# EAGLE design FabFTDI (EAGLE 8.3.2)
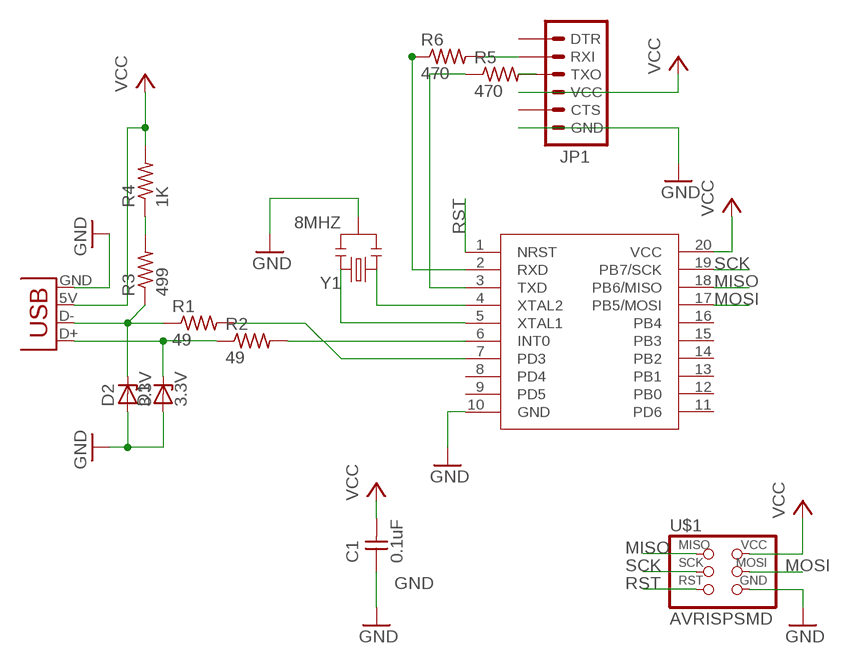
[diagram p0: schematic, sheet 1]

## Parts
C1  0.1uF  UNPOLARIZED_CAPACITOR1206  [1206]
D1  3.3V  ZENER_DIODESOD123  [SOD123]
D2  3.3V  ZENER_DIODESOD123  [SOD123]
JP1  FTDI_CONNECTORSMD  [1X06-SMD]
JP2  USBPCB  [USB_PCB]
R1  49  RESISTOR1206  [1206]
R2  49  RESISTOR1206  [1206]
R3  499  RESISTOR1206  [1206]
R4  1K  RESISTOR1206  [1206]
R5  470  RESISTOR1206  [1206]
R6  470  RESISTOR1206  [1206]
U$1  AVRISPSMD  [2X03SMD]
U$2  ATTINY2313  [SO20W]
Y1  8MHZ  RESONATOR8MHZ  [RESONATOR-SMD]

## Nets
GND: C1.1 D1.ANODE D2.ANODE JP1.6(GND) JP2.GND U$1.6(GND) U$2.10(GND) Y1.2
MISO: U$1.1(MISO) U$2.18(PB6/MISO)
MOSI: U$1.4(MOSI) U$2.17(PB5/MOSI)
N$1: D1.CATHODE JP2.D+ R2.1
N$2: D2.CATHODE JP2.D- R1.1 R3.1
N$3: R2.2 U$2.6(INT0)
N$4: R1.2 U$2.7(PD3)
N$5: R3.2 R4.1
N$7: JP1.2(RXI) R6.2
N$8: JP1.3(TXO) R5.2
N$9: R5.1 U$2.3(TXD)
N$10: R6.1 U$2.2(RXD)
N$11: U$2.4(XTAL2) Y1.1
N$12: U$2.5(XTAL1) Y1.3
RST: U$1.5(RST) U$2.1(NRST)
SCK: U$1.3(SCK) U$2.19(PB7/SCK)
VCC: C1.2 JP1.4(VCC) JP2.5V(VBUS) R4.2 U$1.2(VCC) U$2.20(VCC)
Unconnected: JP1.1(DTR) JP1.5(CTS) U$2.8(PD4) U$2.9(PD5) U$2.11(PD6) U$2.12(PB0) U$2.13(PB1) U$2.14(PB2) U$2.15(PB3) U$2.16(PB4)

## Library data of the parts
C1 = fabPatil:UNPOLARIZED_CAPACITOR: unpolarized_capacitor
D1 D2 = fabPatil:ZENER_DIODE: zener diode
JP1 = fabPatil:FTDI_CONNECTOR: FTDI connector smd
JP2 = fabPatil:USB: USB Connector Connector for USB-microB (orAB), USB-mini, and USB-PCB. For USB-micro use Digikey Part# 609-4052-1-ND (typeB) or 609-4052-1-ND (typeAB).
R1-R6 = fabPatil:RESISTOR
U$1 = fabPatil:AVRISP
U$2 = fabPatil:ATTINY2313
Y1 = fabPatil:RESONATOR: Resonator Small SMD resonator. Used, eg, on the Arduino Pro/ Pro Mini boards. 8MHz- XTAL-08895 16MHz- XTAL-08900; PROD_ID: XTAL-08895

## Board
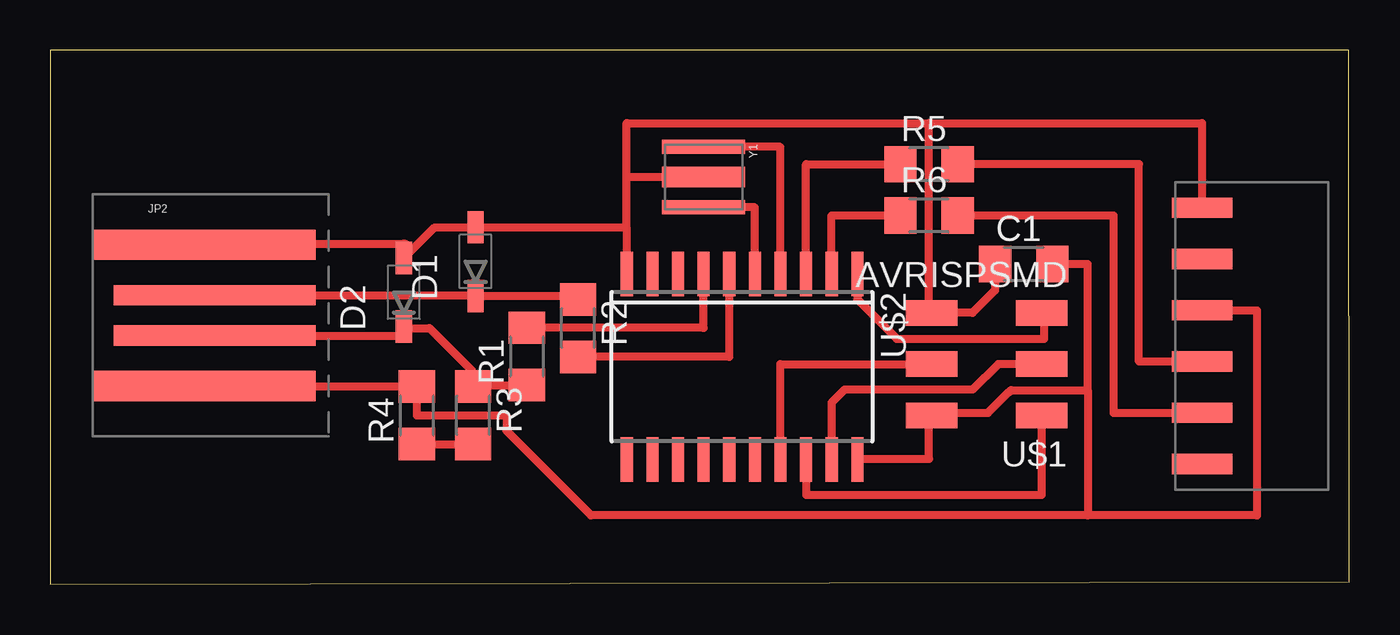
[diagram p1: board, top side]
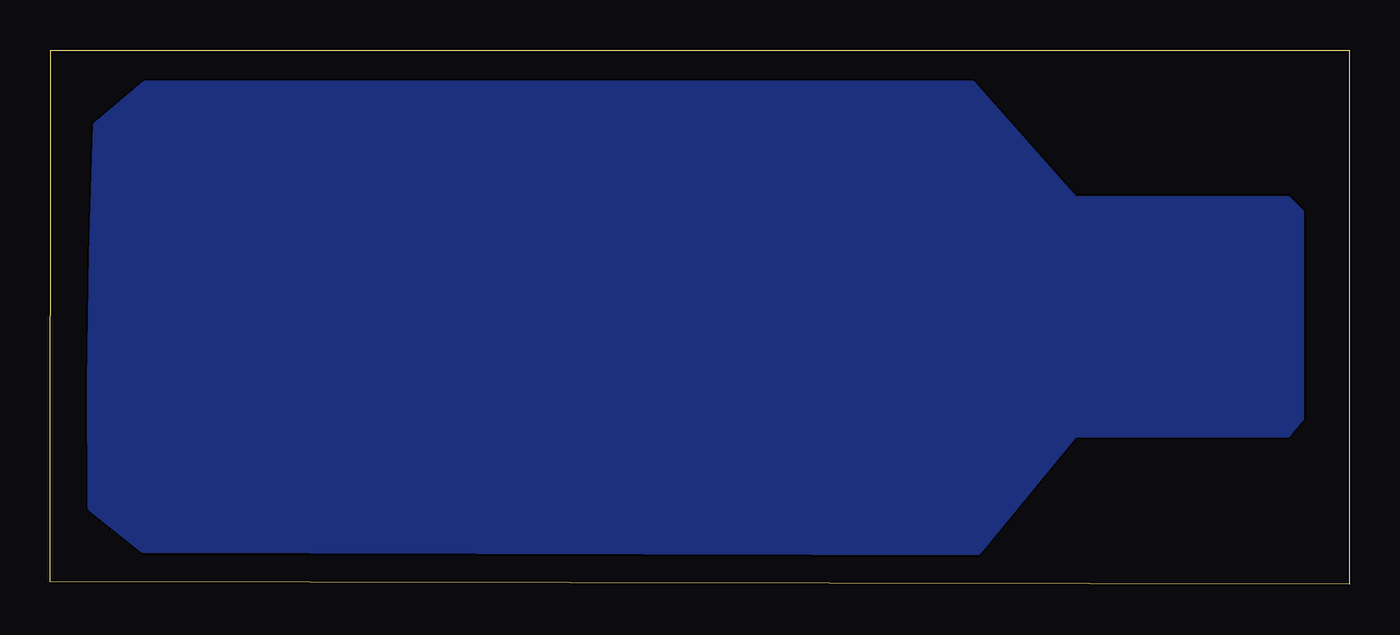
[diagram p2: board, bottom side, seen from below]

Size 64.39 x 26.47 mm. Coordinates in mm from the lower left corner, seen from the top.
Outline: 0,0 64.39,0.13 64.37,26.47 0,26.47 0,0
Copper layers (1*16): Top 0.035mm / dielectric 1.5mm / Bottom 0.035mm
Design rules "Patil": minimum track width 10mil, minimum drill 24mil, track to track 16mil, track to pad 16mil, pad to pad 16mil, via to via 16mil, smd to smd 16mil, copper to edge 40mil, drill to drill 8mil, minimum pad ring 10mil, minimum via ring 8mil, stop-mask expansion 4mil, vias tented up to drill 0mil, thermal gap 10mil

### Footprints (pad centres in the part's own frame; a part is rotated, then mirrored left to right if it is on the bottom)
1206 = smd 1.6 x 1.803: 1 -1.422,0; 2 1.422,0
SOD123 = smd 1.6 x 0.8: ANODE 1.7,0; CATHODE -1.7,0
1X06-SMD = smd 1 x 3: 1 -6.35,-1.35; 2 -3.81,-1.35; 3 -1.27,-1.35; 4 1.27,-1.35; 5 3.81,-1.35; 6 6.35,-1.35
USB_PCB = smd 11 x 1.5: 5V 1.55,-3.5; GND 1.55,3.5 | smd 10 x 1: D+ 2.05,1; D- 2.05,-1
2X03SMD = smd 2.54 x 1.27: 1 -2.54,2.54; 2 2.92,2.54; 3 -2.54,0; 4 2.92,0; 5 -2.54,-2.54; 6 2.92,-2.54
SO20W = smd 0.6 x 2.2: 1 -5.715,-4.6; 2 -4.445,-4.6; 3 -3.175,-4.6; 4 -1.905,-4.6; 5 -0.635,-4.6; 6 0.635,-4.6; 7 1.905,-4.6; 8 3.175,-4.6; 9 4.445,-4.6; 10 5.715,-4.6; 11 5.715,4.6; 12 4.445,4.6; 13 3.175,4.6; 14 1.905,4.6; 15 0.635,4.6; 16 -0.635,4.6; 17 -1.905,4.6; 18 -3.175,4.6; 19 -4.445,4.6; 20 -5.715,4.6
RESONATOR-SMD = smd 0.7 x 4.1: 1 -1.5,0; 3 1.5,0 | smd 1 x 4.1: 2 0,0

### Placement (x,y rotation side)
C1  48.26,15.88 0 top
D1  21.08,16 90 top
D2  17.53,14.48 90 top
JP1  55.75,12.32 90 top
JP2  6.1,13.34 0 top
R1  23.62,11.3 90 top
R2  26.16,12.7 270 top
R3  20.95,8.38 270 top
R4  18.16,8.38 90 top
R5  43.56,20.83 0 top
R6  43.56,18.29 0 top
U$1  46.61,10.92 180 top
U$2  34.29,10.79 180 top
Y1  32.39,20.19 270 top

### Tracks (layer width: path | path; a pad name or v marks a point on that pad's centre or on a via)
GND
  Top 0.406: Y1.2 28.57,20.19 | 28.57,17.65 28.57,20.19 | 28.57,17.65 U$2.10 | JP1.6 57.1,22.86 43.56,22.86 | 43.56,22.86 28.57,22.86 28.57,20.19 | 43.56,22.86 43.56,13.46 U$1.6 45.72,13.46 46.84,14.58 C1.1 | 17.69,16.34 19.05,17.7 D1.ANODE 28.53,17.7 28.57,17.65 | 17.69,16.34 D2.ANODE | JP2.GND arc-90 7.7,16.89 17.53,16.89 arc-90 17.69,16.73 17.69,16.34
MISO
  Top 0.406: U$2.18 37.47,4.45 49.15,4.45 U$1.1
MOSI
  Top 0.406: U$2.17 36.2,10.92 U$1.4
N$1
  Top 0.406: 10.83,14.22 JP2.D+ 21.05,14.34 D1.CATHODE 26.16,14.3 R2.1
N$2
  Top 0.406: R1.1 20.95,9.88 R3.1 20.95,10.54 18.8,12.7 17.65,12.7 | 17.65,12.7 17.6,12.7 D2.CATHODE | JP2.D- 17.29,12.34 17.65,12.7
N$3
  Top 0.406: U$2.6 33.66,11.28 R2.2
N$4
  Top 0.406: U$2.7 32.39,12.7 32.37,12.71 23.62,12.71 R1.2
N$5
  Top 0.406: R4.1 R3.2
N$6
  pour Bottom (no thermals): 2.41,18.41 3.05,19.05 13.59,19.05 18.67,24.77 59.69,24.77 62.1,22.73 arc-3 62.36,3.81 59.82,1.78 18.41,1.65 13.59,7.49 3.05,7.49 2.41,8.26
N$7
  Top 0.406: JP1.2 52.71,8.51 52.71,18.29 R6.2
N$8
  Top 0.406: JP1.3 53.98,11.05 53.98,20.83 R5.2
N$9
  Top 0.406: U$2.3 37.47,20.83 R5.1
N$10
  Top 0.406: U$2.2 38.73,18.29 R6.1
N$11
  Top 0.406: U$2.4 36.2,21.69 Y1.1
N$12
  Top 0.406: U$2.5 34.93,18.69 Y1.3
RST
  Top 0.406: U$2.1 40.01,14.12 41.96,12.17 49.28,12.17 49.28,13.46 U$1.5
SCK
  Top 0.406: U$1.3 46.99,10.92 45.72,9.65 39.37,9.65 38.73,9.02 U$2.19
VCC
  Top 0.406: U$2.20 40.01,6.22 43.56,6.22 43.56,8.38 U$1.2 arc-90 43.82,8.51 46.48,8.51 47.52,9.55 47.55,9.55 47.63,9.63 51.44,9.63 | JP1.4 59.82,13.59 59.82,3.43 51.44,3.43 | C1.2 51.44,15.88 51.44,9.63 | 51.44,9.63 51.44,3.43 | 51.44,3.43 26.8,3.43 22.61,7.62 22.61,8.38 18.16,8.38 R4.2 18.13,9.84 JP2.5V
